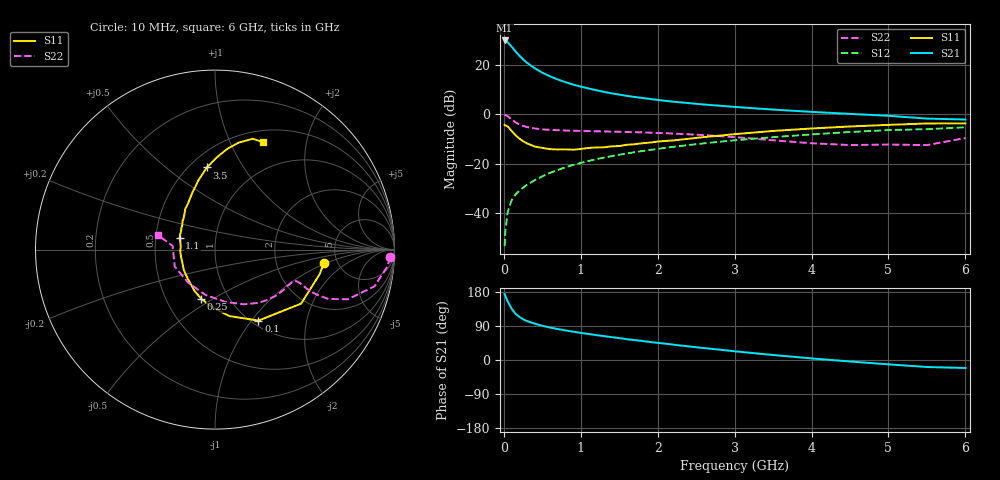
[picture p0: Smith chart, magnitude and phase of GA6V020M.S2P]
! Infineon Technologies  Discrete & RF Semiconductors
! BF775
! Si NPN RF Bipolar Junction Transistor in SOT23
! VCE = 6 V  IC = 20 mA
! Common Emitter S-Parameters:  May  1996
# GHz  S  MA  R  50
!  f  S11  S21  S12  S22
! GHz  MAG  ANG  MAG  ANG  MAG  ANG  MAG  ANG
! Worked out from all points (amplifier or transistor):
!   36 points, 10 MHz to 6 GHz, reference 50 ohm
!   highest |S21| = 30.0 dB at 10 MHz (marker M1)
!   |S21| within 3 dB of that: start of sweep to 113.8 MHz
!   unconditionally stable (mu >= 1): 418.2 MHz to 2.757 GHz
!   at 250 MHz: K = 0.84, MSG = 26.1 dB, |S12| = -29.8 dB
!   at 1.4 GHz: K = 1.10, MAG = 10.8 dB, |S12| = -17.0 dB
!   at 6 GHz: K = 0.91, MSG = 1.6 dB, |S12| = -5.3 dB
!   S11 on the Smith chart (normalised r, x): 10 MHz: 3.92, -0.91; 100 MHz: 1.07, -1.08; 250 MHz: 0.74, -0.44; 1.1 GHz: 0.67, +0.09; 3.5 GHz: 0.61, +0.70; 6 GHz: 0.64, +1.34
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0.01  0.6114 -6.8  31.64 174.2  0.0021 88.2  0.9773 -2.5
0.02  0.5988 -13.3  31.21 168.9  0.0043 83.8  0.9651 -5.6
0.05  0.5664 -32.1  29.14 154.6  0.0104 76.2  0.9114 -13.0
0.1  0.4638 -58.5  23.81 135.9  0.0178 70.1  0.7901 -20.5
0.15  0.3787 -77.9  19.09 122.4  0.0233 65.9  0.6909 -23.5
0.2  0.3236 -92.2  15.65 114.0  0.028 66.4  0.625 -23.9
0.25  0.2847 -105.6  13.05 107.6  0.0324 66.7  0.58 -23.6
0.3  0.2573 -116.2  11.18 102.7  0.037 68.1  0.551 -22.9
0.4  0.2218 -133.4  8.657 96.1  0.0458 69.2  0.5159 -21.7
0.5  0.2078 -146.5  7 90.3  0.0549 70.3  0.4947 -21.3
0.6  0.1961 -157.9  5.916 85.7  0.0648 70.4  0.4845 -21.3
0.7  0.1935 -169.1  5.119 81.7  0.0739 70.7  0.4763 -21.6
0.8  0.1942 -177.6  4.499 78.1  0.0838 70.0  0.4689 -22.2
0.9  0.1911 175.6  4.023 74.7  0.0938 69.9  0.4647 -23.0
1.1  0.2075 161.8  3.354 68.8  0.113 69.1  0.4563 -25.4
1.3  0.2138 152.5  2.858 63.1  0.1319 67.5  0.4488 -27.8
1.6  0.2405 138.7  2.366 54.9  0.1605 64.9  0.4369 -32.4
2.2  0.2948 121.0  1.806 40.6  0.2188 59.2  0.4072 -43.2
3.5  0.4597 95.7  1.247 13.2  0.3437 44.2  0.2973 -78.7
4.5  0.5667 82.9  1.021 -3.9  0.4375 31.2  0.2372 -128.9
5.5  0.6522 71.2  0.819 -18.5  0.4992 15.9  0.2368 175.1
6  0.6556 65.8  0.785 -21.1  0.5459 11.6  0.3301 165.5
